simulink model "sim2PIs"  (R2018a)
settings: Solver=ode15s  StartTime=0.0  StopTime=tsim  RelTol=1e-3
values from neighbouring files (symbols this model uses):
  c0 = 10    [BaseCase.m]    (also in TransformedMVs.m)
  dc = 0*c0    (= 0)    [BaseCase.m]    (also in TransformedMVs.m = 1)
  dM = 0*M0    (= 0)    [BaseCase.m]    (also in TransformedMVs.m)
  dq = 0.1*q0    (= 1)    [BaseCase.m]    (also in TransformedMVs.m = 0)
  Kc_c = 1/k.c*tau.c/(tauC.c+theta)    [BaseCase.m]    (also in TransformedMVs.m)
  Kc_M = 1/k.M/(tauC.M+theta)    [BaseCase.m]    (also in TransformedMVs.m)
  M0 = 1    [BaseCase.m]    (also in TransformedMVs.m = 100; H2P_Turbine_driven.m = param(22); runTD.m = 7.56; H2P_Boiler_driven.m = param(22))
  p = [c1; c2; tau02]    [BaseCase.m]    (also in TransformedMVs.m; Main.m = [N, Fc0, rhoc, rhoh,U,A,cpc,cph]; Main_OL.m = [N, Fc0, rhoc, rhoh,U,A,cpc,cph]; runTestCalcBlk.m = [N, Fc0, rhoc, rhoh,U,A,cpc,cph])
  q0 = 10    [BaseCase.m]    (also in TransformedMVs.m)
  tauI_c = min(tau.c,4*(tauC.c+theta))    [BaseCase.m]    (also in TransformedMVs.m)
  tauI_M = 4*(tauC.M+theta)    [BaseCase.m]    (also in TransformedMVs.m)
  tstep_c = 10    [BaseCase.m]    (also in TransformedMVs.m)
  tstep_d = 100    [BaseCase.m]    (also in TransformedMVs.m)
  tstep_M = 20    [BaseCase.m]    (also in TransformedMVs.m)
  u0 = [q10;q20]    [BaseCase.m]    (also in TransformedMVs.m; runH2Psim.m = [mG0;zV0;mP0;mB0;mA0]; calcblock.m = p(2); testfun.m = 5)
  x0 = [M0;c0]    [BaseCase.m]    (also in TransformedMVs.m; runTD.m = [TE0;TD0;TSh0;MD0; MSh0;w0;TA0;0;0;0;0;0;0;0;0;0]; runBD.m = [TE0;TD0;TSh0;MD0; MSh0;w0;TA0;0;0;0;0;0;0;0;0;0]; runFP.m = [TE0;TD0;TSh0;MD0; MSh0;w0;TA0;0;0;0;0;0;0;0])
undefined symbols (not defined in the file or in its folder): model
libraries: simulink x2

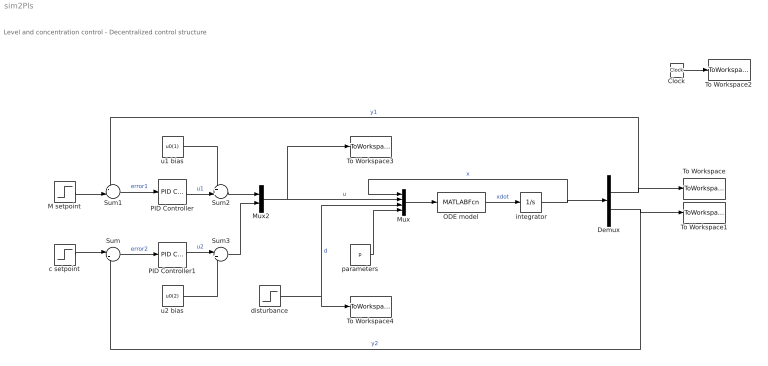
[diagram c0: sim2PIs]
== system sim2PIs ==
  note: Level and concentration control - Decentralized control structure
  " integrator" : Integrator  InitialCondition=x0
  Clock : Clock
  Demux : Demux  Outputs=2
  M setpoint : Step  Time=tstep_M  Before=M0  After=M0+dM  SampleTime=0
  Mux : Mux
  Mux2 : Mux  Inputs=2
  ODE model : MATLABFcn  MATLABFcn=model(u(1:2), u(3:4),u(5),u(6:8))  OutputDimensions=2
  PID Controller : simulink/Continuous/PID Controller  Controller=PI  TimeDomain=Continuous-time  SampleTime=-1  IntegratorMethod=Forward Euler  FilterMethod=Forward Euler  Form=Ideal  UseFilter=on  ControllerParametersSource=internal  P=Kc_M  I=1/tauI_M  D=0  N=100  InitialConditionSource=internal  InitialConditionForIntegrator=0  InitialConditionForFilter=0  ExternalReset=none  LimitOutput=off  UpperSaturationLimit=inf  LowerSaturationLimit=-inf  LinearizeAsGain=on  AntiWindupMode=none  Kb=1  TrackingMode=off  Kt=1  PParamMin=[]  PParamMax=[]  IParamMin=[]  IParamMax=[]  DParamMin=[]  DParamMax=[]  NParamMin=[]  NParamMax=[]  KbParamMin=[]  KbParamMax=[]  KtParamMin=[]  KtParamMax=[]  POutMin=[]  POutMax=[]  IOutMin=[]  IOutMax=[]  DOutMin=[]  DOutMax=[]  NOutMin=[]  NOutMax=[]  KbOutMin=[]  KbOutMax=[]  KtOutMin=[]  KtOutMax=[]  IntegratorOutMin=[]  IntegratorOutMax=[]  FilterOutMin=[]  FilterOutMax=[]  SumOutMin=[]  SumOutMax=[]  SumI1OutMin=[]  SumI1OutMax=[]  SumI2OutMin=[]  SumI2OutMax=[]  SumI3OutMin=[]  SumI3OutMax=[]  SumDOutMin=[]  SumDOutMax=[]  SaturationOutMin=[]  SaturationOutMax=[]  IntegratorContinuousStateAttributes=''  IntegratorStateMustResolveToSignalObject=off  IntegratorRTWStateStorageClass=Auto  FilterContinuousStateAttributes=''  FilterStateMustResolveToSignalObject=off  FilterRTWStateStorageClass=Auto  DifferentiatorICPrevScaledInput=0  DifferentiatorOutMin=[]  DifferentiatorOutMax=[]  FilterDiffOutCoefMin=[]  FilterDiffOutCoefMax=[]  SumDenOutMin=[]  SumDenOutMax=[]  SumNumOutMin=[]  SumNumOutMax=[]  ReciprocalOutMin=[]  ReciprocalOutMax=[]  DivideOutMin=[]  DivideOutMax=[]  TunerSelectOption=Transfer Function Based (PID Tuner App)
  PID Controller1 : simulink/Continuous/PID Controller  Controller=PI  TimeDomain=Continuous-time  SampleTime=-1  IntegratorMethod=Forward Euler  FilterMethod=Forward Euler  Form=Ideal  UseFilter=on  ControllerParametersSource=internal  P=Kc_c  I=1/tauI_c  D=0  N=100  InitialConditionSource=internal  InitialConditionForIntegrator=0  InitialConditionForFilter=0  ExternalReset=none  LimitOutput=off  UpperSaturationLimit=inf  LowerSaturationLimit=-inf  LinearizeAsGain=on  AntiWindupMode=none  Kb=1  TrackingMode=off  Kt=1  PParamMin=[]  PParamMax=[]  IParamMin=[]  IParamMax=[]  DParamMin=[]  DParamMax=[]  NParamMin=[]  NParamMax=[]  KbParamMin=[]  KbParamMax=[]  KtParamMin=[]  KtParamMax=[]  POutMin=[]  POutMax=[]  IOutMin=[]  IOutMax=[]  DOutMin=[]  DOutMax=[]  NOutMin=[]  NOutMax=[]  KbOutMin=[]  KbOutMax=[]  KtOutMin=[]  KtOutMax=[]  IntegratorOutMin=[]  IntegratorOutMax=[]  FilterOutMin=[]  FilterOutMax=[]  SumOutMin=[]  SumOutMax=[]  SumI1OutMin=[]  SumI1OutMax=[]  SumI2OutMin=[]  SumI2OutMax=[]  SumI3OutMin=[]  SumI3OutMax=[]  SumDOutMin=[]  SumDOutMax=[]  SaturationOutMin=[]  SaturationOutMax=[]  IntegratorContinuousStateAttributes=''  IntegratorStateMustResolveToSignalObject=off  IntegratorRTWStateStorageClass=Auto  FilterContinuousStateAttributes=''  FilterStateMustResolveToSignalObject=off  FilterRTWStateStorageClass=Auto  DifferentiatorICPrevScaledInput=0  DifferentiatorOutMin=[]  DifferentiatorOutMax=[]  FilterDiffOutCoefMin=[]  FilterDiffOutCoefMax=[]  SumDenOutMin=[]  SumDenOutMax=[]  SumNumOutMin=[]  SumNumOutMax=[]  ReciprocalOutMin=[]  ReciprocalOutMax=[]  DivideOutMin=[]  DivideOutMax=[]  TunerSelectOption=Transfer Function Based (PID Tuner App)
  Sum : Sum  Inputs=|+-
  Sum1 : Sum  Inputs=-+|
  Sum2 : Sum  Inputs=++|
  Sum3 : Sum  Inputs=|++
  To Workspace : ToWorkspace  VariableName=M  SampleTime=-1
  To Workspace1 : ToWorkspace  VariableName=c  SampleTime=-1
  To Workspace2 : ToWorkspace  VariableName=time  SampleTime=-1
  To Workspace3 : ToWorkspace  VariableName=u  SampleTime=-1
  To Workspace4 : ToWorkspace  VariableName=d  SampleTime=-1
  c setpoint : Step  Time=tstep_c  Before=c0  After=c0+dc  SampleTime=0
  disturbance : Step  Time=tstep_d  Before=q0  After=q0+dq  SampleTime=0
  parameters : Constant  Value=p
  u1 bias : Constant  Value=u0(1)
  u2 bias : Constant  Value=u0(2)
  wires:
  ODE model/1 -> " integrator"/1  "xdot"
  Demux/1 -> To Workspace/1, Sum1/1  "y1"
  Mux/1 -> ODE model/1
  Clock/1 -> To Workspace2/1
  Sum/1 -> PID Controller1/1  "error2"
  c setpoint/1 -> Sum/1
  Sum1/1 -> PID Controller/1  "error1"
  M setpoint/1 -> Sum1/2
  PID Controller/1 -> Sum2/2  "u1"
  PID Controller1/1 -> Sum3/1  "u2"
  u1 bias/1 -> Sum2/1
  u2 bias/1 -> Sum3/2
  Sum2/1 -> Mux2/1
  Sum3/1 -> Mux2/2
  Demux/2 -> Sum/2, To Workspace1/1  "y2"
  disturbance/1 -> Mux/3, To Workspace4/1  "d"
  " integrator"/1 -> Demux/1, Mux/1  "x"
  Mux2/1 -> To Workspace3/1, Mux/2  "u"
  parameters/1 -> Mux/4
